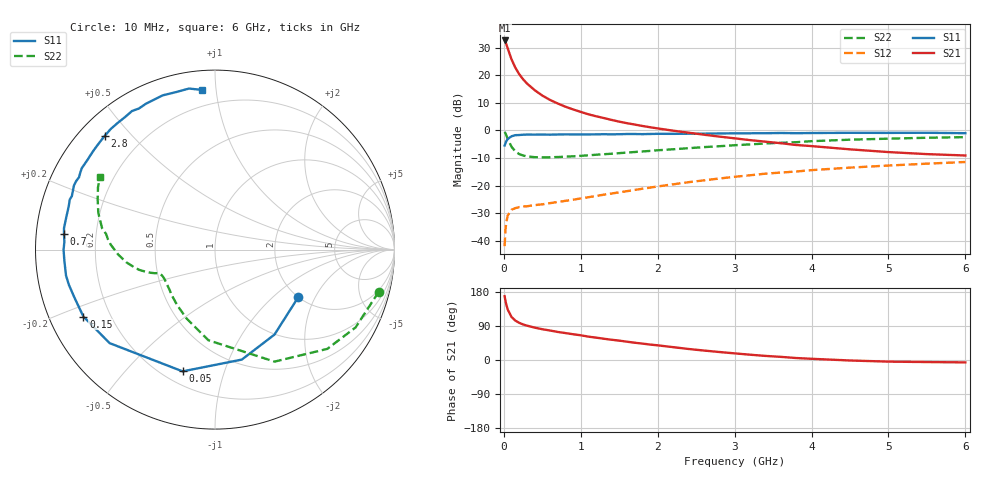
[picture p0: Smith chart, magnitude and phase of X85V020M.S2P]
! SIEMENS Small Signal Semiconductors
! BFP136W
! Si NPN RF Bipolar Junction Transistor in SOT343
! VCE = 5 V  IC = 20 mA
! Common Emitter S-Parameters:  September  1994
# GHz  S  MA  R  50
!  f  S11  S21  S12  S22
! GHz  MAG  ANG  MAG  ANG  MAG  ANG  MAG  ANG
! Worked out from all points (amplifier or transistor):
!   40 points, 10 MHz to 6 GHz, reference 50 ohm
!   highest |S21| = 32.6 dB at 10 MHz (marker M1)
!   |S21| within 3 dB of that: start of sweep to 51.79 MHz
!   unconditionally stable (mu >= 1): 882.2 MHz to 2.758 GHz
!   at 200 MHz: K = 0.32, MSG = 24.1 dB, |S12| = -27.8 dB
!   at 1.5 GHz: K = 1.16, MAG = 10.3 dB, |S12| = -22.4 dB
!   at 6 GHz: K = 0.98, MSG = 1.2 dB, |S12| = -11.4 dB
!   S11 on the Smith chart (normalised r, x): 10 MHz: 1.99, -1.48; 50 MHz: 0.27, -0.73; 150 MHz: 0.10, -0.24; 700 MHz: 0.08, +0.05; 2.8 GHz: 0.07, +0.42; 6 GHz: 0.10, +0.92
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0.01  0.5343 -29.8  42.83 168.4  0.008 76.3  0.9424 -14.4
0.02  0.5779 -55.0  40.05 157.4  0.0151 68.5  0.8952 -29.0
0.03  0.6308 -76.3  37.5 148.1  0.0208 60.1  0.8349 -41.5
0.05  0.702 -104.9  30.82 133.2  0.0287 46.6  0.7068 -62.0
0.1  0.785 -138.4  19.44 113.5  0.0366 31.6  0.5063 -94.2
0.15  0.8227 -153.0  13.73 103.9  0.0391 26.9  0.415 -112.5
0.2  0.8271 -160.9  10.46 98.0  0.0409 24.6  0.3737 -124.5
0.25  0.8373 -166.4  8.486 93.8  0.0419 24.4  0.3521 -132.5
0.3  0.8425 -170.1  7.125 90.7  0.0423 24.5  0.3387 -138.3
0.4  0.8416 -175.9  5.383 85.5  0.0444 26.3  0.3284 -145.7
0.5  0.8437 -179.9  4.298 81.2  0.0459 28.9  0.3257 -150.3
0.6  0.8404 177.1  3.579 77.8  0.0482 31.3  0.3271 -152.9
0.7  0.8457 174.1  3.084 74.1  0.0506 34.5  0.3302 -154.6
0.9  0.8483 169.9  2.409 68.0  0.0556 38.8  0.3402 -157.1
1.1  0.8486 165.0  1.963 61.6  0.0617 42.6  0.355 -158.3
1.6  0.8631 155.6  1.355 48.4  0.0794 49.1  0.3973 -161.7
2.2  0.8687 145.0  0.992 33.9  0.1056 51.4  0.4561 -167.1
2.8  0.883 134.0  0.775 21.1  0.1346 49.9  0.5184 -174.5
3.2  0.89 127.4  0.669 14.0  0.1542 47.3  0.5594 -179.9
4.5  0.9074 108.7  0.455 -1.3  0.2123 36.4  0.6813 162.6
5.5  0.9089 99.2  0.373 -5.4  0.2503 28.1  0.7384 152.0
6  0.8929 94.7  0.352 -6.3  0.2686 23.5  0.7579 147.7
